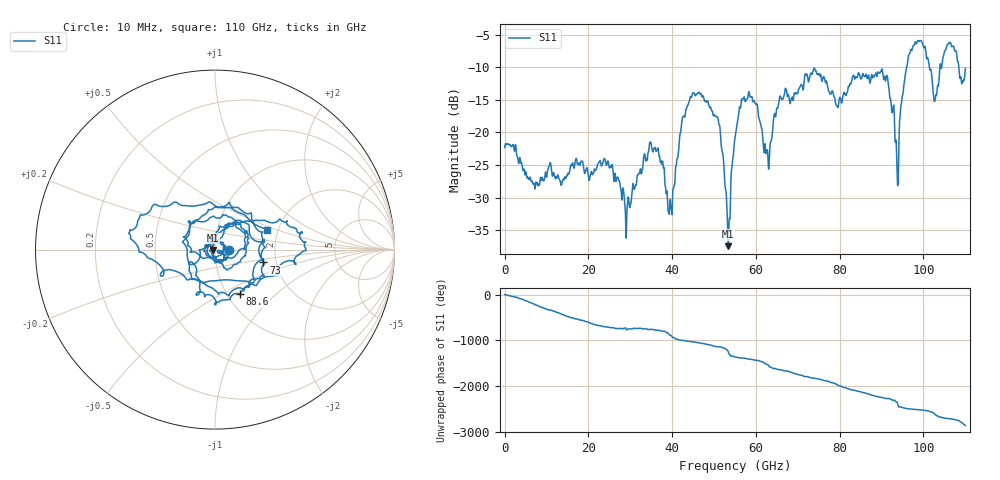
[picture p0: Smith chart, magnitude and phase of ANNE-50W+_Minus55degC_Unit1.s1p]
!Mini-Circuits Laboratory
!S-Parameters
!S1P File: Measurement
!Model: ANNE-50W+
!No.: Unit# 1 (U1_-55°C)
!Run / Lot / Date Code: QN2409253 /  / 2409
!Fixture: N/A
!Network Analyzer: PNA-X N5242B;  Serial number: 74314
!Pin Outs: PORT<1> = pin<1>
!TEST CONDITIONS: Z:50 OHM SYSTEM, INPUT POWER = 0dBm, TEMP:25°C
!F-F adapter to 1FT F-M cable on Port 2 head. 1mm 1 PORT SmartCal
!Date: 9/5/2024 at 12:57:31 PM
# Hz  S  dB  R  50
!Frequency  S11 dB  S11 Deg
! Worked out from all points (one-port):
!   2208 points, 10 MHz to 110 GHz, reference 50 ohm
!   lowest |S11| = -37.4 dB at 53.4 GHz (marker M1), VSWR 1.03, Z = 48.7 - j0.196 ohm
!   |S11| at or under -10 dB: start of sweep to 95.97 GHz; 101.4 GHz to 103.9 GHz (2.509 GHz wide, 2.44 % of centre); 108.4 GHz to end of sweep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
!   S11 on the Smith chart (normalised r, x): 10 MHz: 1.17, -0.00; 73 GHz: 1.71, -0.27; 88.6 GHz: 1.15, -0.62; 110 GHz: 1.75, +0.43
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1e7  -22.32 -0.3
1.38e10  -27.44 -77.6
2.755e10  -27.79 -18.5
2.94e10  -30.42 -39.5
3.51e10  -22.23 -37.7
3.95e10  -30.29 -165.6
4.13e10  -23.93 104.3
4.385e10  -15.66 59.3
4.695e10  -14.12 18.5
5.1e10  -18.01 -60.2
5.34e10  -37.44 -171.4
5.505e10  -20.68 77.3
5.865e10  -14.56 27.2
6.28e10  -23.03 -90.5
6.55e10  -15.14 159.0
6.88e10  -14.87 90.2
7.3e10  -11.09 -14.8
7.66e10  -12.37 -81.3
7.98e10  -15.23 169.5
8.255e10  -12.57 88.3
8.86e10  -10.88 -60.7
9.13e10  -11.28 -111.6
9.37e10  -26.15 164.3
9.63e10  -8.74 24.3
1e11  -6.86 -4.9
1.0275e11  -15.11 -96.6
1.0605e11  -6.27 169.4
1.1e11  -10.18 21.0
